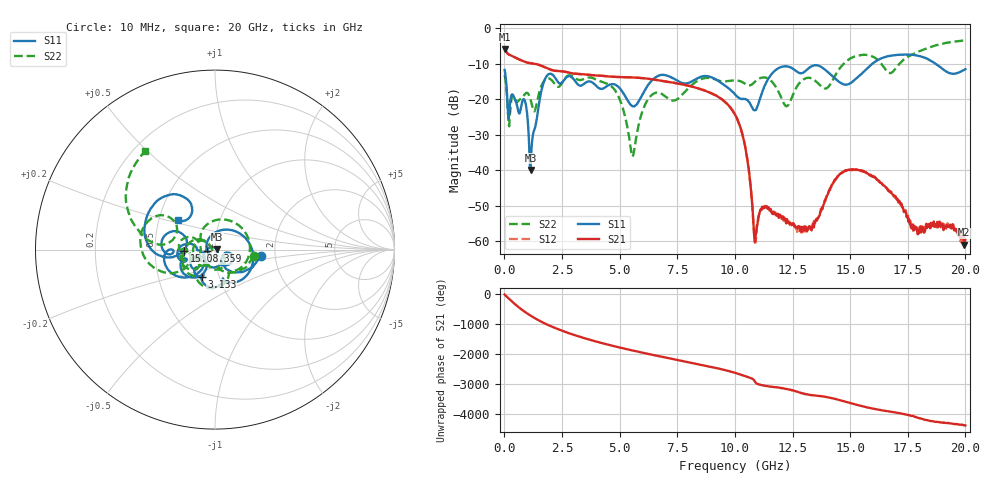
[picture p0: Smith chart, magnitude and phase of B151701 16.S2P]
!  2-Port S-parameters saved by WinCal
! VAR MeasName=S-Parameters (CALIBRATED_DATA) read from VNA (N5244A)
! VAR MeasDate=2015-12-24 19:10:00
! VAR NAME=B151701 16
! VAR FILENAME=B151701 16.S2P
! VAR DATE=2015-12-24 19:10:00
! VAR PHYS_PORTS=1,3
# Hz S DB R 50
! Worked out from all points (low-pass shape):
!   801 points, 10 MHz to 20 GHz, reference 50 ohm
!   highest |S21| = -5.83 dB at 10 MHz (marker M1); lowest = -61.0 dB at 19.95 GHz (marker M2)
!   |S21| within 3 dB of the highest: start of sweep to 644.5 MHz
!   lowest |S11| = -40.0 dB at 1.134 GHz (marker M3), VSWR 1.02, Z = 50.9 + j0.41 ohm
!   |S11| at or under -10 dB: start of sweep to 15.97 GHz; 18.7 GHz to end of sweep
!   |S22| runs from -36.2 to -3.5 dB; largest |S21 - S12| = 0.0022
!   S11 on the Smith chart (normalised r, x): 10 MHz: 1.68, -0.13; 1.359 GHz: 0.92, -0.01; 3.133 GHz: 0.82, -0.26; 15.08 GHz: 0.70, -0.01; 20 GHz: 0.63, +0.22
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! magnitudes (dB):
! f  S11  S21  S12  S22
! 10 MHz  -11.8  -5.8  -5.8  -13.2
! 209.9 MHz  -24.1  -7.5  -7.5  -27.7
! 884.6 MHz  -20.4  -9.5  -9.5  -18.6
! 1.134 GHz  -40.0  -9.9  -9.9  -20.1
! 1.359 GHz  -27.2  -10.1  -10.1  -22.5
! 1.884 GHz  -13.1  -11.4  -11.4  -14.2
! 3.133 GHz  -15.5  -12.9  -12.9  -14.3
! 3.358 GHz  -16.1  -13.0  -13.0  -14.6
! 4.783 GHz  -15.9  -13.7  -13.7  -17.4
! 5.557 GHz  -22.0  -13.9  -13.9  -36.2
! 6.682 GHz  -13.4  -14.7  -14.7  -18.2
! 10.01 GHz  -18.6  -24.3  -24.3  -14.7
! 10.48 GHz  -20.1  -34.6  -34.6  -15.8
! 10.88 GHz  -23.1  -60.1  -60.5  -15.0
! 11.28 GHz  -16.4  -50.7  -50.5  -13.9
! 12.25 GHz  -10.8  -53.8  -53.9  -22.0
! 13.35 GHz  -10.7  -56.1  -56.5  -14.2
! 15.08 GHz  -15.2  -39.9  -39.8  -8.3
! 16.68 GHz  -7.8  -45.9  -45.8  -12.6
! 17.85 GHz  -7.6  -56.3  -56.4  -7.0
! 19.95 GHz  -11.7  -61.0  -60.4  -3.5
! 20 GHz  -11.6  -59.5  -61.1  -3.5
